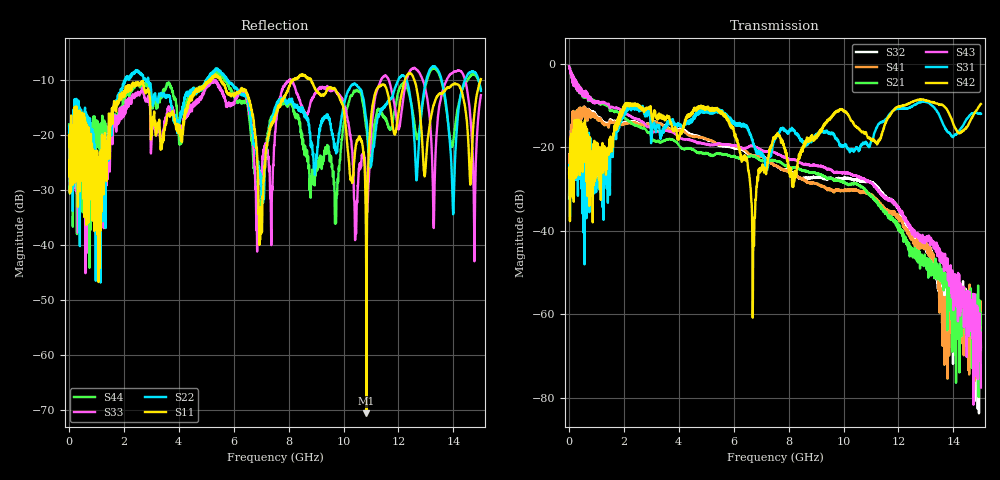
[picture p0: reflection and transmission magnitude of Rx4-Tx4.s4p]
! FILE: N:\QM 2007\Prüfprotokolle\Highspeed\Konfektionierte Ltg\L45593-D106\D30\8216\0002  kpl\IL  mit Chris Boards\Rx4-Tx4.s4p
# MHz S DB R 50.00
! FREQ  S11  S12  S13  S14
!  S21  S22  S23  S24
!  S31  S32  S33  S34
!  S41  S42  S43  S44
!  DB  ANG  DB  ANG  DB  ANG  DB  ANG
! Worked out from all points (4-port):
!   2999 points, 10 MHz to 15 GHz, reference 50 ohm
!   strongest paths, dB at 10 MHz, 3.755 GHz, 7.505 GHz, 11.26 GHz, 15 GHz:
!     S42: -26.3, -15.0, -18.1, -18.9, -9.7
!     S31: -25.0, -13.4, -18.1, -14.7, -12.0
!     S43: -0.6, -16.4, -21.3, -30.3, -77.6
!     S21: -0.6, -18.2, -23.1, -33.6, -68.9
!     S41: -31.5, -15.9, -24.3, -32.9, -62.2
!     S32: -32.3, -15.9, -24.4, -29.8, -67.8
!   lowest |S11| = -70.7 dB at 10.84 GHz (marker M1), VSWR 1.00, Z = 50 - j0.0148 ohm
!   |S11| at or under -10 dB: start of sweep to 5.125 GHz; 5.533 GHz to 8.153 GHz (2.619 GHz wide, 38.3 % of centre); 8.819 GHz to 12.24 GHz (3.424 GHz wide, 32.5 % of centre)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
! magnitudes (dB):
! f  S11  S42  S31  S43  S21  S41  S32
! 10 MHz  -20.2  -26.3  -25.0  -0.6  -0.6  -31.5  -32.3
! 5.375 GHz  -9.3  -11.0  -11.3  -19.4  -21.6  -19.2  -19.3
! 6.97 GHz  -37.1  -25.6  -21.3  -20.6  -23.2  -22.1  -22.1
! 8.545 GHz  -9.3  -20.1  -18.8  -24.1  -25.6  -27.7  -27.5
! 10.84 GHz  -70.7  -16.8  -19.2  -27.9  -30.6  -31.1  -28.2
! 11.25 GHz  -11.4  -18.9  -14.8  -30.4  -33.3  -32.9  -29.8
! 15 GHz  -9.9  -9.7  -12.0  -77.6  -68.9  -62.2  -67.8
